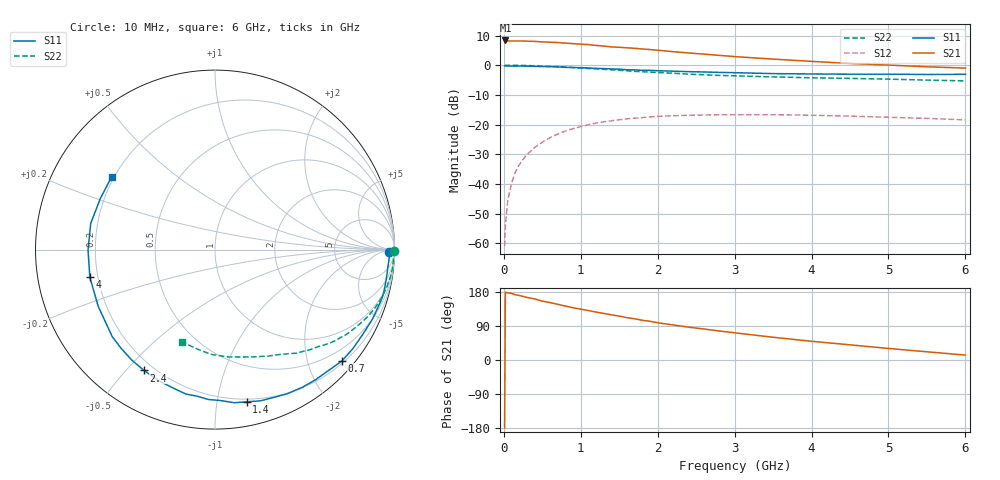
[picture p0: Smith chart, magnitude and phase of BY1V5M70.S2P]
! SIEMENS Small Signal Semiconductors
! BFY420
! Si NPN RF SIEGET Grounded Emitter Transistor in MICRO-X
! VCE = 1.5 V  IC = 0.7 mA
! Common Emitter S-Parameters:  October  1996
# GHz  S  MA  R  50
!  f  S11  S21  S12  S22
! GHz  MAG  ANG  MAG  ANG  MAG  ANG  MAG  ANG
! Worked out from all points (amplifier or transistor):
!   36 points, 10 MHz to 6 GHz, reference 50 ohm
!   highest |S21| = 8.4 dB at 20 MHz (marker M1)
!   |S21| within 3 dB of that: start of sweep to 1.867 GHz
!   unconditionally stable (mu >= 1): 4.71 GHz to end of sweep
!   at 250 MHz: K = 0.03, MSG = 19.9 dB, |S12| = -31.7 dB
!   at 1.4 GHz: K = 0.20, MSG = 12.4 dB, |S12| = -18.7 dB
!   at 6 GHz: K = 1.38, MAG = 5.0 dB, |S12| = -18.4 dB
!   S11 on the Smith chart (normalised r, x): 10 MHz: 56, -27; 700 MHz: 0.24, -2.64; 1.4 GHz: 0.18, -1.21; 2.4 GHz: 0.16, -0.56; 4 GHz: 0.17, -0.11; 6 GHz: 0.19, +0.31
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0.01  0.9715 -0.8  2.605 -179.3  0.0009 98.4  0.9993 -0.3
0.02  0.9748 -1.4  2.616 178.7  0.002 83.0  0.9999 -0.6
0.05  0.9712 -3.1  2.57 177.1  0.0052 90.6  0.9987 -1.5
0.1  0.9682 -6.1  2.562 175.7  0.0104 87.2  0.9957 -3.0
0.15  0.968 -9.0  2.56 172.0  0.0159 82.9  0.9953 -4.6
0.2  0.9688 -12.1  2.562 170.3  0.0211 82.2  0.9949 -6.1
0.4  0.9588 -24.0  2.523 161.2  0.0413 74.6  0.9804 -12.1
0.5  0.9493 -29.8  2.474 155.4  0.0507 71.2  0.9702 -15.0
0.7  0.941 -41.2  2.413 147.0  0.0693 64.2  0.9458 -20.6
0.9  0.9162 -52.4  2.31 137.9  0.0857 56.7  0.9156 -25.8
1.1  0.8988 -63.3  2.227 130.4  0.0997 50.2  0.8844 -30.7
1.4  0.8662 -78.3  2.036 119.2  0.1161 41.4  0.8389 -37.3
1.6  0.8411 -88.1  1.968 111.7  0.1254 35.8  0.8065 -41.3
1.8  0.8227 -96.8  1.881 104.8  0.1316 30.9  0.7785 -44.9
2.2  0.7952 -113.1  1.694 92.5  0.1415 21.9  0.7344 -51.8
2.4  0.7809 -120.4  1.612 86.7  0.1438 18.4  0.709 -54.9
2.8  0.759 -133.6  1.468 76.6  0.147 11.4  0.6746 -60.6
3.5  0.7235 -154.1  1.269 60.0  0.1474 1.9  0.6363 -69.9
4  0.7141 -167.6  1.163 49.4  0.1439 -3.4  0.615 -76.7
4.5  0.7073 -179.9  1.073 40.0  0.1394 -7.8  0.6009 -83.8
5.5  0.6994 156.0  0.941 21.6  0.1274 -13.0  0.5624 -100.3
6  0.7044 144.9  0.896 13.0  0.1204 -13.4  0.5455 -109.6
